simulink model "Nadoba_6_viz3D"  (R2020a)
settings: Solver=VariableStepAuto  StartTime=0.0  StopTime=inf  RelTol=1e-3  EnableMultiTasking=on
libraries: vrlib x5

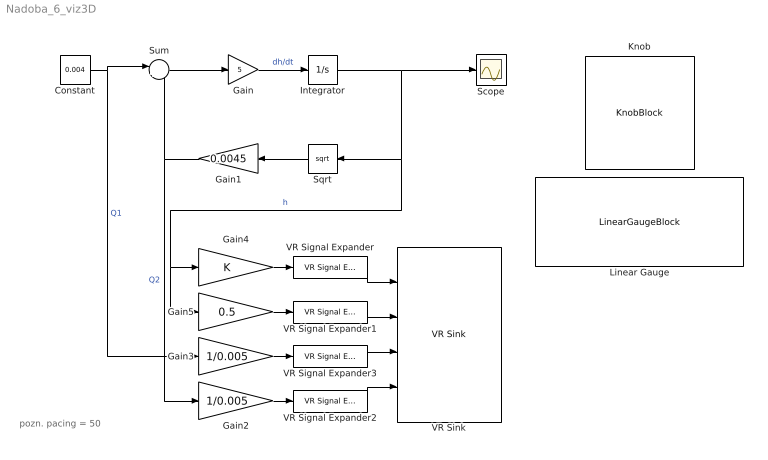
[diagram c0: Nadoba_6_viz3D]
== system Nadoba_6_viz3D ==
  note: pozn. pacing = 50
  Constant : Constant  Value=0.004
  Gain : Gain  Gain=5
  Gain1 : Gain  Gain=0.0045
  Gain2 : Gain  Gain=1/0.005
  Gain3 : Gain  Gain=1/0.005
  Gain4 : Gain
  Gain5 : Gain  Gain=0.5
  Integrator : Integrator  LimitOutput=on  UpperSaturationLimit=1
  Knob : KnobBlock  ScaleMax=0.005
  Linear Gauge : LinearGaugeBlock  ScaleMax=2
  Scope : Scope
  Sqrt : Sqrt
  Sum : Sum  Inputs=|+-
  VR Signal Expander : vrlib/VR Signal Expander  outwidth=3  outidx=[2]
  VR Signal Expander1 : vrlib/VR Signal Expander  outwidth=3  outidx=[2]
  VR Signal Expander2 : vrlib/VR Signal Expander  outwidth=3  outidx=[1 3]
  VR Signal Expander3 : vrlib/VR Signal Expander  outwidth=3  outidx=[1 3]
  VR Sink : vrlib/VR Sink  InstantiateOnLoad=on  SampleTime=1  ViewEnable=on  RemoteChange=off  RemoteView=on  FieldsWritten=Voda.scale.3.1.1.double#Voda.translation.3.1.1.double#Pritok.scale.3.1.1.double#Vytok.scale.3.1.1.double  WorldFileName=Nadrz_v1.wrl  AutoView=on  VideoDimensions=[]  AllowVariableSize=off  FigureProperties={'Position', 'Name', 'Viewpoint', 'CameraBound', 'CameraDirection', 'CameraPosition', 'CameraUpVector', 'ZoomFactor', 'Antialiasing', 'Headlight', 'Lighting', 'NavPanel', 'Sound', 'StatusBar', 'Stereo3D', 'Stereo3DCameraOffset', 'Stereo3DHIT', 'ToolBar', 'Textures', 'Transparency', 'Triad', 'Wireframe', 'NavZones', 'NavMode', 'NavSpeed', 'CaptureFileFormat', 'CaptureFileName', 'Record2DCompressMet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
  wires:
  Gain/1 -> Integrator/1  "dh/dt"
  Constant/1 -> Gain3/1, Sum/1  "Q1"
  Integrator/1 -> Scope/1, Sqrt/1, Gain4/1, Gain5/1  "h"
  Sqrt/1 -> Gain1/1
  Gain1/1 -> Sum/2, Gain2/1  "Q2"
  Sum/1 -> Gain/1
  VR Signal Expander/1 -> VR Sink/1
  VR Signal Expander3/1 -> VR Sink/3
  VR Signal Expander2/1 -> VR Sink/4
  VR Signal Expander1/1 -> VR Sink/2
  Gain3/1 -> VR Signal Expander3/1
  Gain5/1 -> VR Signal Expander1/1
  Gain2/1 -> VR Signal Expander2/1
  Gain4/1 -> VR Signal Expander/1
